(* Logix 5000 AddOnInstructionDefinition export Banner_IOL_Analog_Converter_Param_v4; software revision 33.00 *)

TYPE Banner_Analog_Converter_Port_Mirroringv4 :
STRUCT
   Mirroring_Output_Enable : SINT;   // 0 = Disabled, 1 = Enabled.
   Mirroring_Input_Port_Selection : SINT;   // 0 = Analog In 1, 1 = Analog In 2.
END_STRUCT
END_TYPE

TYPE Banner_Analog_Converter_RD_v4 :   // All of the read parameters for a S15C-I, S15C-U, R45-K-IQ, R45-K-UQ, R45C-KUU-UUQ, or R45C-KII-IIQ.
STRUCT
   Master_Cycle_Time : INT;
   Min_Cycle_Time : INT;
   M_Sequence_Capability : INT;
   IO_Link_Version_ID : INT;
   Process_Data_Input_Length : INT;
   Process_Data_Output_Length : INT;
   Combined_Vendor_ID : DINT;   // IO-Link Vendor ID
   Vendor_ID1 : INT;
   Vendor_ID2 : INT;
   Combined_Device_ID : DINT;   // IO-Link Device ID
   Device_ID1 : INT;
   Device_ID2 : INT;
   Device_ID3 : INT;
   Serial_Number : STRING;
   Product_Name : STRING;
   All_Time_Run_Time : DINT;   // Current All Time Run Timer.
   Model_Type : SINT;   // 0 = Voltage, 1 = Current
   MDC : Banner_MDC_Descriptor_v4[3];   // Array 0 not used. Array 1 is used for all models. Array 2 used for R45C Analog Double models.
END_STRUCT
END_TYPE

TYPE Banner_Analog_Converter_v4 :   // All of the parameters for a S15C-I, S15C-U, R45-K-IQ, R45-K-UQ, R45C-KUU-UUQ, or R45C-KII-IIQ.
STRUCT
   Initial_Global_Read : BOOL;   // Determines if all of the IO-Link data has been read into the PLC yet
   Command : INT;   // Value placed in here will activate a read or write to a specifc IO-Link Index
   Read : Banner_Analog_Converter_RD_v4;   // Read Only Data
   Write : Banner_Analog_Converter_WD_v4;   // Write Data
   Archive : Banner_Analog_Converter_WD_v4;   // Archive Data
   Reset : BOOL;   // Resets AOI. This will force a complete parameter read of the sensor.
END_STRUCT
END_TYPE

TYPE Banner_Analog_Converter_VSC_v4 :   // Vendor Specific Configuration data.
STRUCT
   PDI_Configuration : INT;   // 0 = Analog Value, 1 = Digital Measuring Sensor
   IOL_Filter_Time : DINT;   // Time to average IOL Process Data management between updates.
   PDO_Outside_Valid_Range : SINT;   // R45C-IU models only. 0 = Hold, 1 = Low, 2 = High.
   SSC1_PDO_Outside_Valid_Range : SINT;   // R45C Double Analog Models. 0 = Hold, 1 = Low, 2 = High.
   SSC2_PDO_Outside_Valid_Range : SINT;   // R45C Double Analog Models. 0 = Hold, 1 = Low, 2 = High.
   Secondary_Output_Function : SINT;   // R45C Double Analog Models. 0 = Disabled, 1 = Pulse Frequency Modulation.
   PFM_Input_Port : SINT;   // R45C Double Analog Models. 0 = Analog In1, 1 = Analog In 2.
END_STRUCT
END_TYPE

TYPE Banner_Analog_Converter_WD_v4 :   // UDT that stores the Write Data for a S15C-I, S15C-U, R45-K-IQ, R45-K-UQ, R45C-KUU-UUQ, or R45C-KII-IIQ.
STRUCT
   System_Command : INT;   // See IODD file for list of commands that can be activated via the System Command interface
   Parameter_Access_Lock : SINT;   // Write access to all parameters is prohibited while value is 1. Only this parameter can be adjusted when value is 1.
   Data_Storage_Lock : SINT;   // Automatic data storage is disabled when this value is equal to 1. Read access is not affected.
   Local_Parameterization_Lock : SINT;   // Parameterization via local control elements on device is disabled.
   Local_User_Interface_Lock : SINT;   // Operation of local user interface is disabled.
   BDC_Parameters : Banner_BDC_Parameters_v4[3];
   Port_Mirroring : Banner_Analog_Converter_Port_Mirroringv4[3];   // Only Double Analog Models.
   Resetable_Run_Time : DINT;   // Current Resetable Run Timer.
   VSC : Banner_Analog_Converter_VSC_v4;   // Vendor Specifc Configuration.
   All_Time_Run_Time_Event_Time : DINT;   // Time before an Event is generated. 0 = disable all-time event.
   Resetable_Run_Time_Event_Time : DINT;   // Time before an Event is generated. 0 = disable run time event.
   Pulse_Frequency : Banner_Pulse_Frequency_v4;
END_STRUCT
END_TYPE

TYPE Banner_BDC_Parameters_v4 :
STRUCT
   Setpoint_SP1 : DINT;
   Setpoint_SP2 : DINT;
   Switchpoint_Logic : SINT;   // 0 = Light Operate - Discrete Output is On while target detected.
   BDC_Mode : SINT;   // 2 = Window Mode. Defines how the binary switching information is created depending on Setpoint parameters and the current measurement value.
   Hysteresis : INT;   // Hysteresis value for the switchpoint.
END_STRUCT
END_TYPE

TYPE Banner_IOL_Port_v4 :   // UDT that has all of the data items necessary to communicate with a specific Port on a IO-Link Master
STRUCT
   Port_Controlled : INT;   // Each bit represents a port on an IO-Link Master. Set to 1 to tell AOI to control that port.
   Port_Activate : INT;   // Each bit represents a port on an IO-Link Master. When ON that port will process any commands in queue.
   Port_Read : INT;   // Each bit represents a port on an IO-Link Master. Used to determine when device AOI has requested a Read command.
   Port_Write : INT;   // Each bit represents a port on an IO-Link Master. Used to determine when device AOI has requested a Write command.
   Port_RW_Complete : INT;   // Each bit represents a port on an IO-Link Master. Tells device AOI that Read or Write request has been completed.
   Port_Device_Read : INT;
   Data_Transfer : SINT[190];   // Array to transfer data from IO-Master to device AOIs.
END_STRUCT
END_TYPE

TYPE Banner_MDC_Descriptor_v4 :
STRUCT
   Lower_Limit : DINT;
   Upper_Limit : DINT;
   Unit : DINT;   // 1209 = A, 1240 = V
   Scale : DINT;   // 260 = microAmps, 253 = microVolts
END_STRUCT
END_TYPE

TYPE Banner_Pulse_Frequency_v4 :   // Data items related to Pulse Frequency.
STRUCT
   Near_Frequency : DINT;   // 100 to 45000. Frequency corresponding to a target at the near limit of the sensing range.
   Far_Frequency : DINT;   // 100 to 45000. Frequency corresponding to a target at the far limit of the sensing range.
   Pulse_Frequenc_LOS : DINT;   // 50 to 45000. The frequency used to indicate loss of signal.
END_STRUCT
END_TYPE

ADD_ON_INSTRUCTION Banner_IOL_Analog_Converter_Param_v4   (* revision 4.0, vendor Banner Engineering *)
// AOI to read and write parameter data to an IO-Link S15C-I, S15C-U, R45-K-IQ, R45-K-UQ, R45C-KUU-UUQ, or R45C-KII-IIQ.
VAR_IN_OUT
   Converter : Banner_Analog_Converter_v4; {required}
   Port_Data : Banner_IOL_Port_v4; {required}
END_VAR
VAR_INPUT
   Port : DINT; {required}
   Type : DINT; {required}   // 0 for S15C U/I models. 1 for R45C U/I models. 2 for R45C UU/II double analog models.
END_VAR
VAR
   Local_Control : DINT; {access None}
   Global_Read_Command_Value : INT; {access None}
   Global_Write_Command_Value : INT; {access None}
   Error_Generated : BOOL; {access None}
   Command_Being_Processed : BOOL; {access None}
   Index_Write_Inprocess : INT; {access None}
   Index_Write_Control : INT; {access None}
   Update_Archive : BOOL; {access None}
   Inprocess_Index : DINT; {access None}
   Index : DINT; {access None}
   Index2 : DINT; {access None}
   Index3 : DINT; {access None}
END_VAR

ROUTINE Logic   (* ladder *)
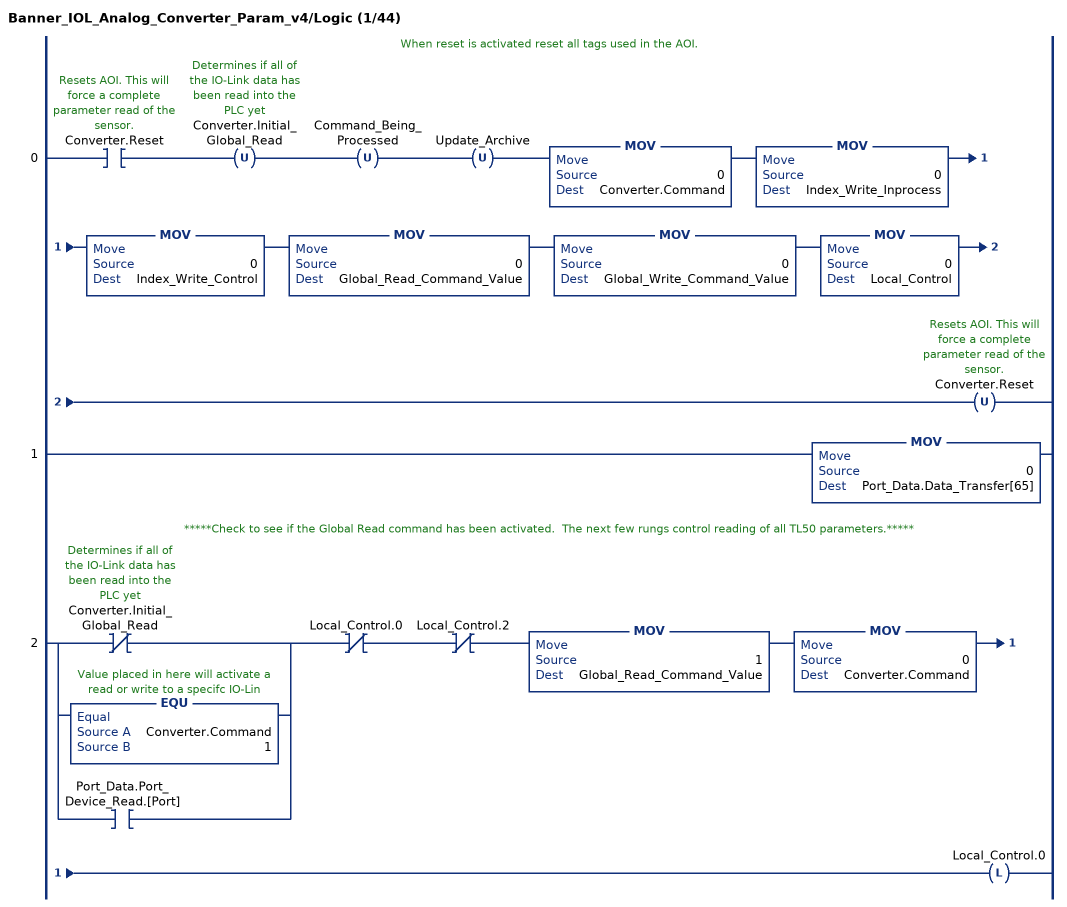
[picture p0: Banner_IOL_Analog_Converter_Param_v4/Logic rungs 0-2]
   // When reset is activated reset all tags used in the AOI.
   0: XIC(Converter.Reset)OTU(Converter.Initial_Global_Read)OTU(Command_Being_Processed)OTU(Update_Archive)MOV(0,Converter.Command)MOV(0,Index_Write_Inprocess)MOV(0,Index_Write_Control)MOV(0,Global_Read_Command_Value)MOV(0,Global_Write_Command_Value)MOV(0,Local_Control)OTU(Converter.Reset);
   1: MOV(0,Port_Data.Data_Transfer[65]);
   // *****Check to see if the Global Read command has been activated.  The next few rungs control reading of all TL50 parameters.*****
   2: [XIO(Converter.Initial_Global_Read) ,EQU(Converter.Command,1) ,XIC(Port_Data.Port_Device_Read.[Port]) ]XIO(Local_Control.0)XIO(Local_Control.2)MOV(1,Global_Read_Command_Value)MOV(0,Converter.Command)OTL(Local_Control.0);
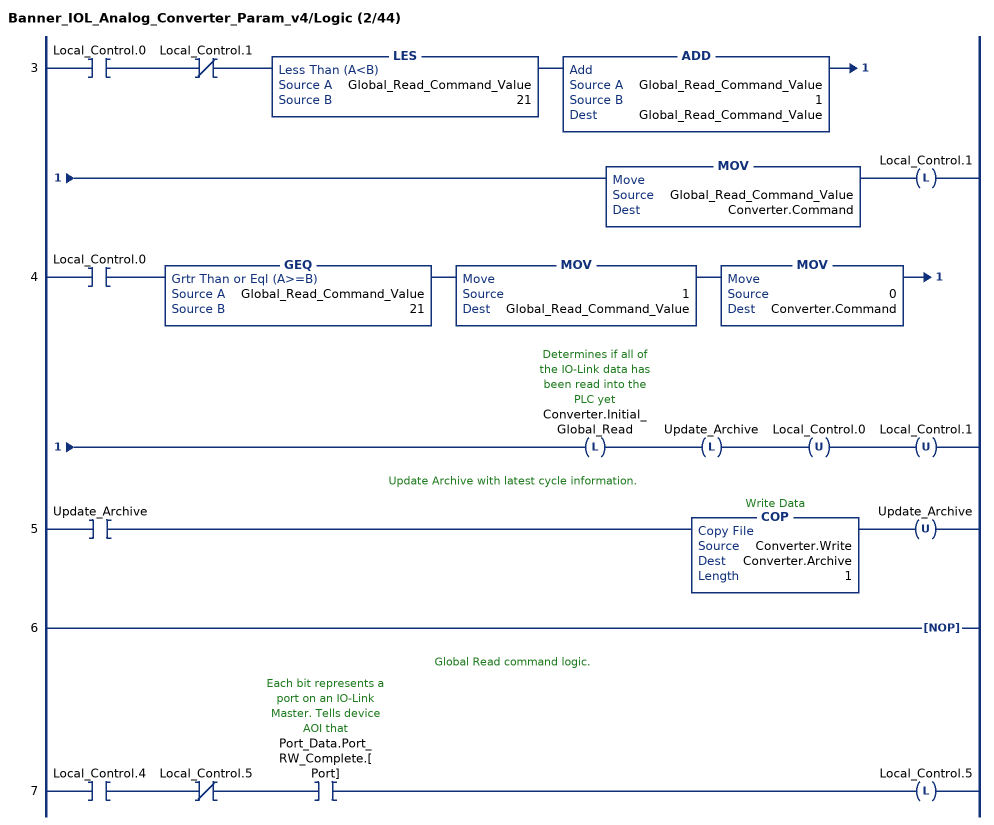
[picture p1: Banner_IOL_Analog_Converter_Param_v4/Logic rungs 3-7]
   3: XIC(Local_Control.0)XIO(Local_Control.1)LES(Global_Read_Command_Value,21)ADD(Global_Read_Command_Value,1,Global_Read_Command_Value)MOV(Global_Read_Command_Value,Converter.Command)OTL(Local_Control.1);
   4: XIC(Local_Control.0)GEQ(Global_Read_Command_Value,21)MOV(1,Global_Read_Command_Value)MOV(0,Converter.Command)OTL(Converter.Initial_Global_Read)OTL(Update_Archive)OTU(Local_Control.0)OTU(Local_Control.1);
   // Update Archive with latest cycle information.
   5: XIC(Update_Archive)COP(Converter.Write,Converter.Archive,1)OTU(Update_Archive);
   6: NOP();
   // Global Read command logic.
   7: XIC(Local_Control.4)XIO(Local_Control.5)XIC(Port_Data.Port_RW_Complete.[Port])OTL(Local_Control.5);
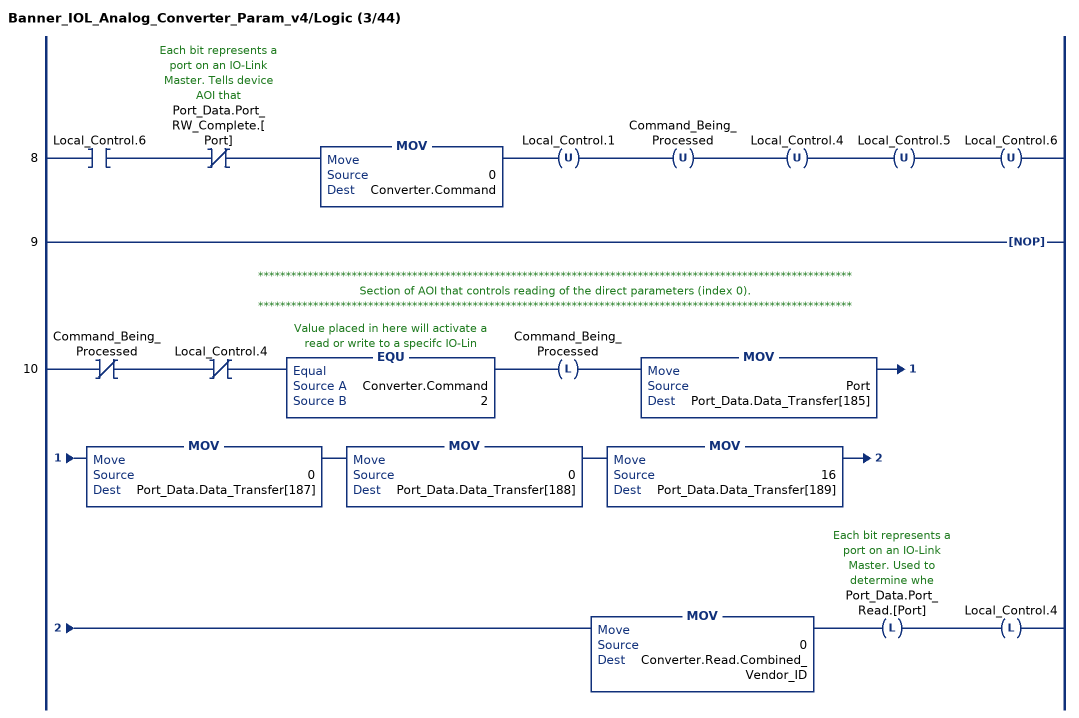
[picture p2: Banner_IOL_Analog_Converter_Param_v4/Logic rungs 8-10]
   8: XIC(Local_Control.6)XIO(Port_Data.Port_RW_Complete.[Port])MOV(0,Converter.Command)OTU(Local_Control.1)OTU(Command_Being_Processed)OTU(Local_Control.4)OTU(Local_Control.5)OTU(Local_Control.6);
   9: NOP();
   // ************************************************************************************************************
   // Section of AOI that controls reading of the direct parameters (index 0).
   // ************************************************************************************************************
   10: XIO(Command_Being_Processed)XIO(Local_Control.4)EQU(Converter.Command,2)OTL(Command_Being_Processed)MOV(Port,Port_Data.Data_Transfer[185])MOV(0,Port_Data.Data_Transfer[187])MOV(0,Port_Data.Data_Transfer[188])MOV(16,Port_Data.Data_Transfer[189])MOV(0,Converter.Read.Combined_Vendor_ID)OTL(Port_Data.Port_Read.[Port])OTL(Local_Control.4);
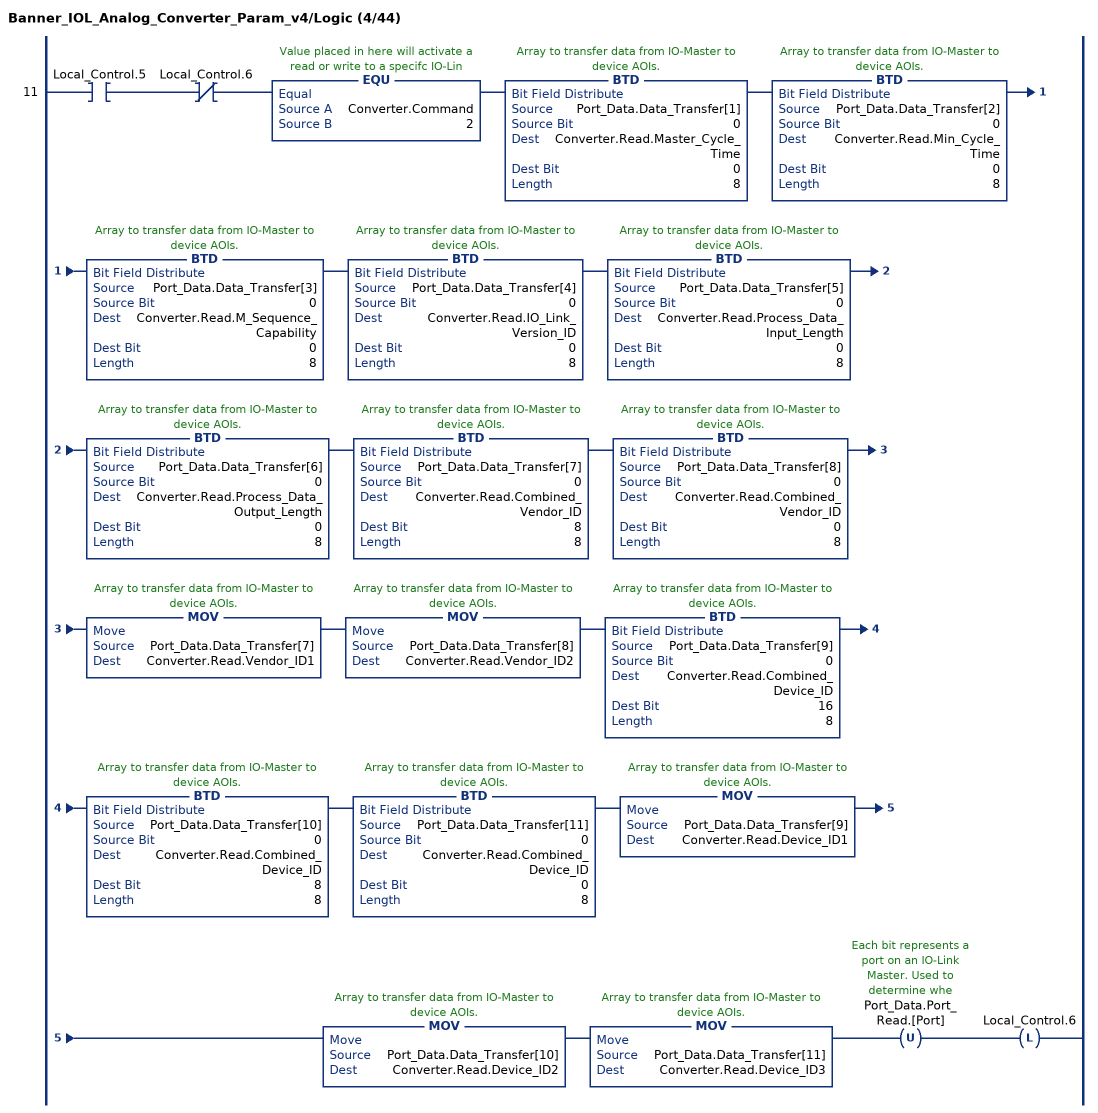
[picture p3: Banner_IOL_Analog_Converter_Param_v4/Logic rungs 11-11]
   11: XIC(Local_Control.5)XIO(Local_Control.6)EQU(Converter.Command,2)BTD(Port_Data.Data_Transfer[1],0,Converter.Read.Master_Cycle_Time,0,8)BTD(Port_Data.Data_Transfer[2],0,Converter.Read.Min_Cycle_Time,0,8)BTD(Port_Data.Data_Transfer[3],0,Converter.Read.M_Sequence_Capability,0,8)BTD(Port_Data.Data_Transfer[4],0,Converter.Read.IO_Link_Version_ID,0,8)BTD(Port_Data.Data_Transfer[5],0,Converter.Read.Process_Data_Input_Length,0,8)BTD(Port_Data.Data_Transfer[6],0,Converter.Read.Process_Data_Output_Length,0,8)BTD(Port_Data.Data_Transfer[7],0,Converter.Read.Combined_Vendor_ID,8,8)BTD(Port_Data.Data_Transfer[8],0,Converter.Read.Combined_Vendor_ID,0,8)MOV(Port_Data.Data_Transfer[7],Converter.Read.Vendor_ID1)MOV(Port_Data.Data_Transfer[8],Converter.Read.Vendor_ID2)BTD(Port_Data.Data_Transfer[9],0,Converter.Read.Combined_Device_ID,16,8)BTD(Port_Data.Data_Transfer[10],0,Converter.Read.Combined_Device_ID,8,8)BTD(Port_Data.Data_Transfer[11],0,Converter.Read.Combined_Device_ID,0,8)MOV(Port_Data.Data_Transfer[9],Converter.Read.Device_ID1)MOV(Port_Data.Data_Transfer[10],Converter.Read.Device_ID2)MOV(Port_Data.Data_Transfer[11],Converter.Read.Device_ID3)OTU(Port_Data.Port_Read.[Port])OTL(Local_Control.6);
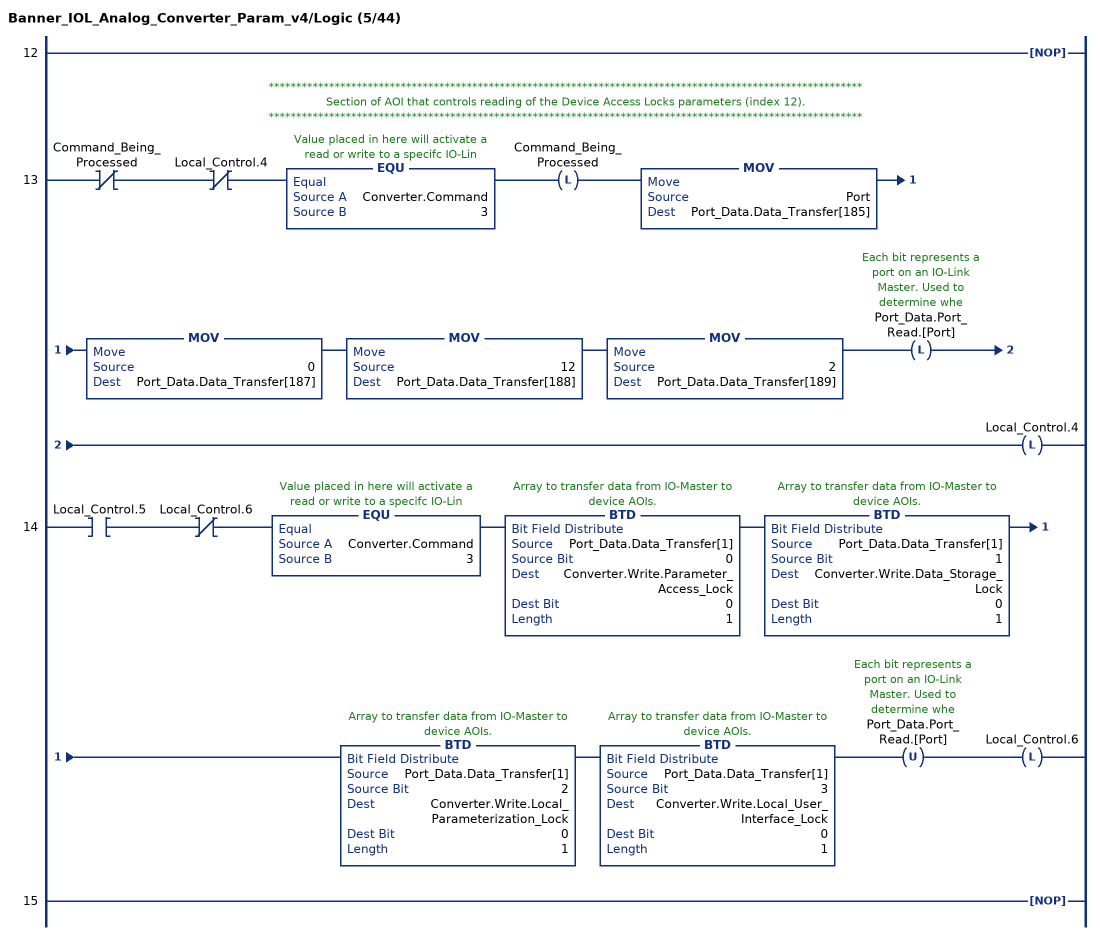
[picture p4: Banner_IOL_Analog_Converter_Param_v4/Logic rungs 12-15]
   12: NOP();
   // ************************************************************************************************************
   // Section of AOI that controls reading of the Device Access Locks parameters (index 12).
   // ************************************************************************************************************
   13: XIO(Command_Being_Processed)XIO(Local_Control.4)EQU(Converter.Command,3)OTL(Command_Being_Processed)MOV(Port,Port_Data.Data_Transfer[185])MOV(0,Port_Data.Data_Transfer[187])MOV(12,Port_Data.Data_Transfer[188])MOV(2,Port_Data.Data_Transfer[189])OTL(Port_Data.Port_Read.[Port])OTL(Local_Control.4);
   14: XIC(Local_Control.5)XIO(Local_Control.6)EQU(Converter.Command,3)BTD(Port_Data.Data_Transfer[1],0,Converter.Write.Parameter_Access_Lock,0,1)BTD(Port_Data.Data_Transfer[1],1,Converter.Write.Data_Storage_Lock,0,1)BTD(Port_Data.Data_Transfer[1],2,Converter.Write.Local_Parameterization_Lock,0,1)BTD(Port_Data.Data_Transfer[1],3,Converter.Write.Local_User_Interface_Lock,0,1)OTU(Port_Data.Port_Read.[Port])OTL(Local_Control.6);
   15: NOP();
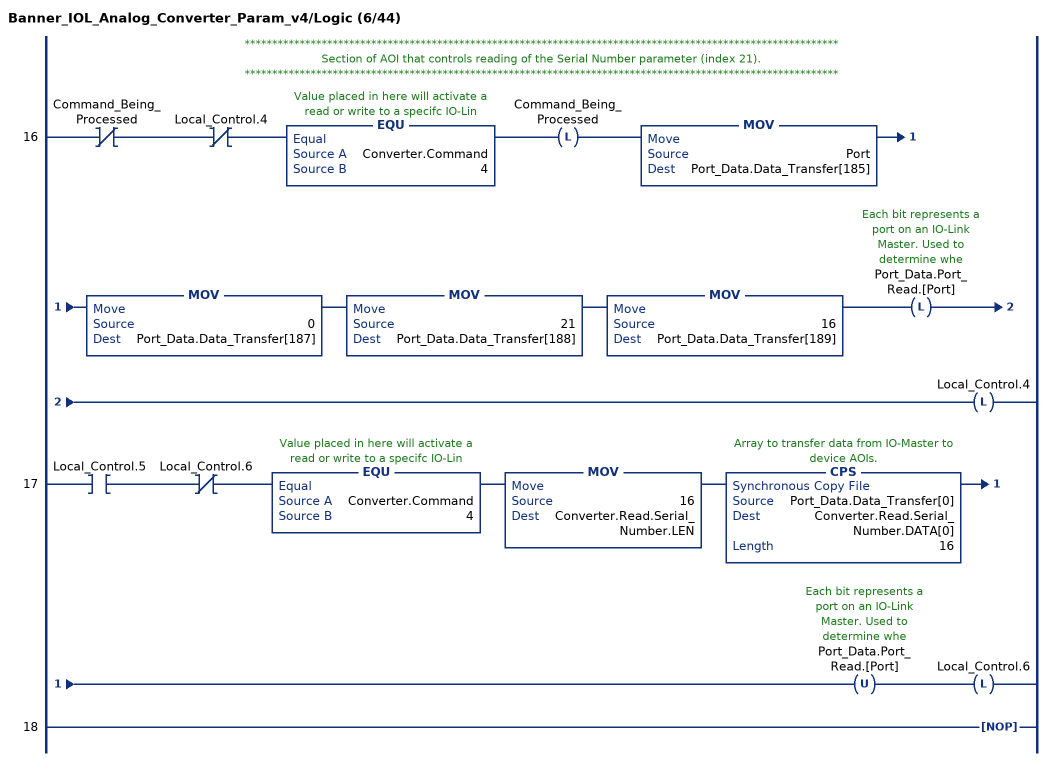
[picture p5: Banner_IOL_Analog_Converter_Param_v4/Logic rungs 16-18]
   // ************************************************************************************************************
   // Section of AOI that controls reading of the Serial Number parameter (index 21).
   // ************************************************************************************************************
   16: XIO(Command_Being_Processed)XIO(Local_Control.4)EQU(Converter.Command,4)OTL(Command_Being_Processed)MOV(Port,Port_Data.Data_Transfer[185])MOV(0,Port_Data.Data_Transfer[187])MOV(21,Port_Data.Data_Transfer[188])MOV(16,Port_Data.Data_Transfer[189])OTL(Port_Data.Port_Read.[Port])OTL(Local_Control.4);
   17: XIC(Local_Control.5)XIO(Local_Control.6)EQU(Converter.Command,4)MOV(16,Converter.Read.Serial_Number.LEN)CPS(Port_Data.Data_Transfer[0],Converter.Read.Serial_Number.DATA[0],16)OTU(Port_Data.Port_Read.[Port])OTL(Local_Control.6);
   18: NOP();
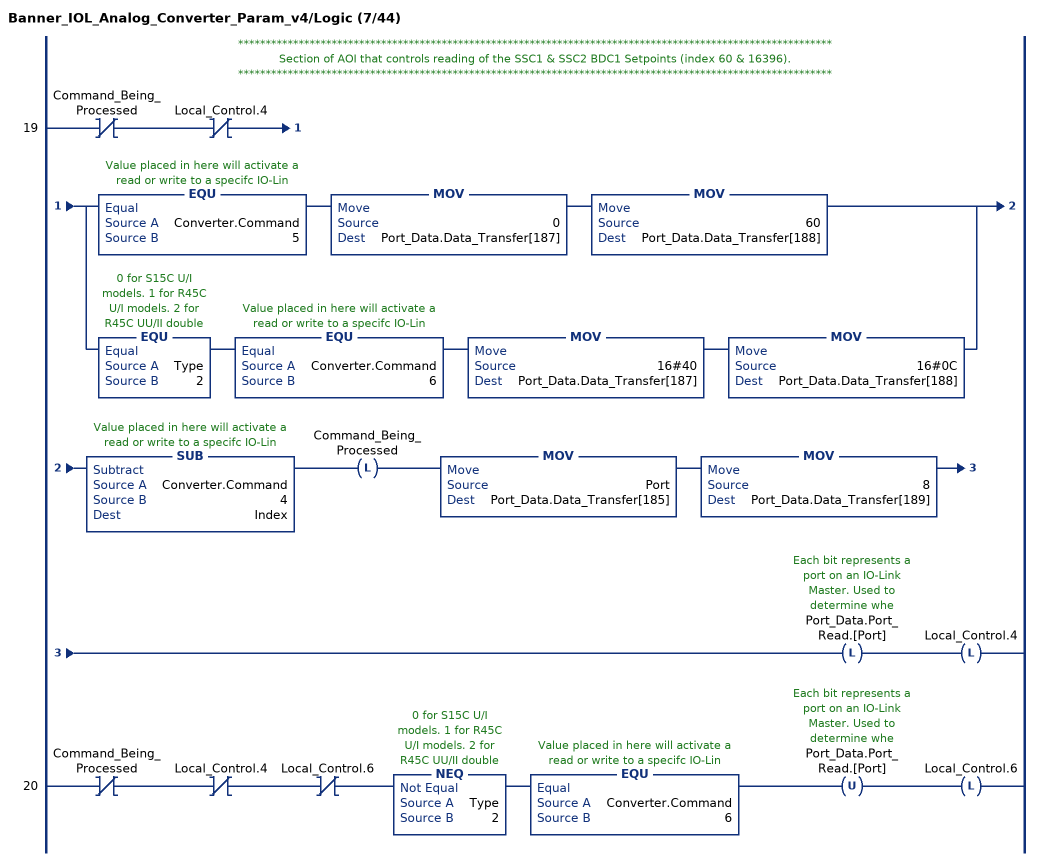
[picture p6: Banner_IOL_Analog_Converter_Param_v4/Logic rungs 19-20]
   // ************************************************************************************************************
   // Section of AOI that controls reading of the SSC1 & SSC2 BDC1 Setpoints (index 60 & 16396).
   // ************************************************************************************************************
   19: XIO(Command_Being_Processed)XIO(Local_Control.4)[EQU(Converter.Command,5) MOV(0,Port_Data.Data_Transfer[187]) MOV(60,Port_Data.Data_Transfer[188]) ,EQU(Type,2) EQU(Converter.Command,6) MOV(16#40,Port_Data.Data_Transfer[187]) MOV(16#0C,Port_Data.Data_Transfer[188]) ]SUB(Converter.Command,4,Index)OTL(Command_Being_Processed)MOV(Port,Port_Data.Data_Transfer[185])MOV(8,Port_Data.Data_Transfer[189])OTL(Port_Data.Port_Read.[Port])OTL(Local_Control.4);
   20: XIO(Command_Being_Processed)XIO(Local_Control.4)XIO(Local_Control.6)NEQ(Type,2)EQU(Converter.Command,6)OTU(Port_Data.Port_Read.[Port])OTL(Local_Control.6);
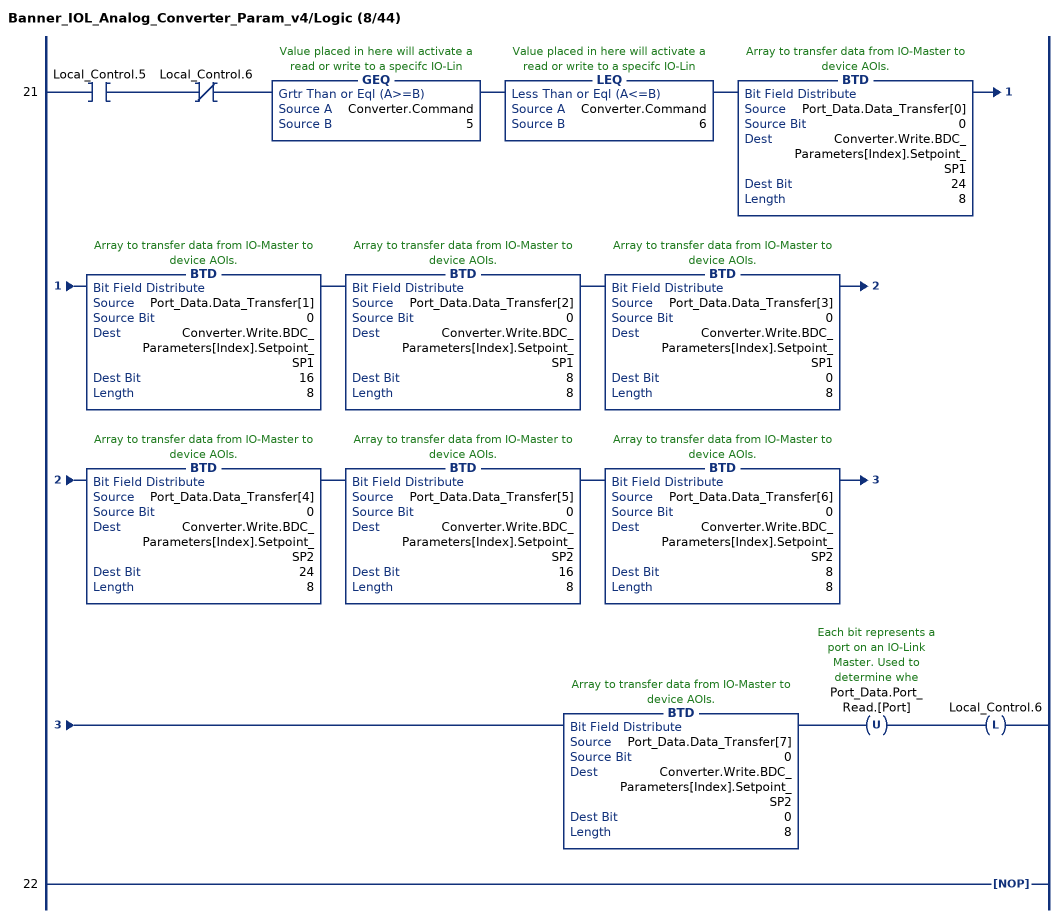
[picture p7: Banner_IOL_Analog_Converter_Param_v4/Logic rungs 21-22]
   21: XIC(Local_Control.5)XIO(Local_Control.6)GEQ(Converter.Command,5)LEQ(Converter.Command,6)BTD(Port_Data.Data_Transfer[0],0,Converter.Write.BDC_Parameters[Index].Setpoint_SP1,24,8)BTD(Port_Data.Data_Transfer[1],0,Converter.Write.BDC_Parameters[Index].Setpoint_SP1,16,8)BTD(Port_Data.Data_Transfer[2],0,Converter.Write.BDC_Parameters[Index].Setpoint_SP1,8,8)BTD(Port_Data.Data_Transfer[3],0,Converter.Write.BDC_Parameters[Index].Setpoint_SP1,0,8)BTD(Port_Data.Data_Transfer[4],0,Converter.Write.BDC_Parameters[Index].Setpoint_SP2,24,8)BTD(Port_Data.Data_Transfer[5],0,Converter.Write.BDC_Parameters[Index].Setpoint_SP2,16,8)BTD(Port_Data.Data_Transfer[6],0,Converter.Write.BDC_Parameters[Index].Setpoint_SP2,8,8)BTD(Port_Data.Data_Transfer[7],0,Converter.Write.BDC_Parameters[Index].Setpoint_SP2,0,8)OTU(Port_Data.Port_Read.[Port])OTL(Local_Control.6);
   22: NOP();
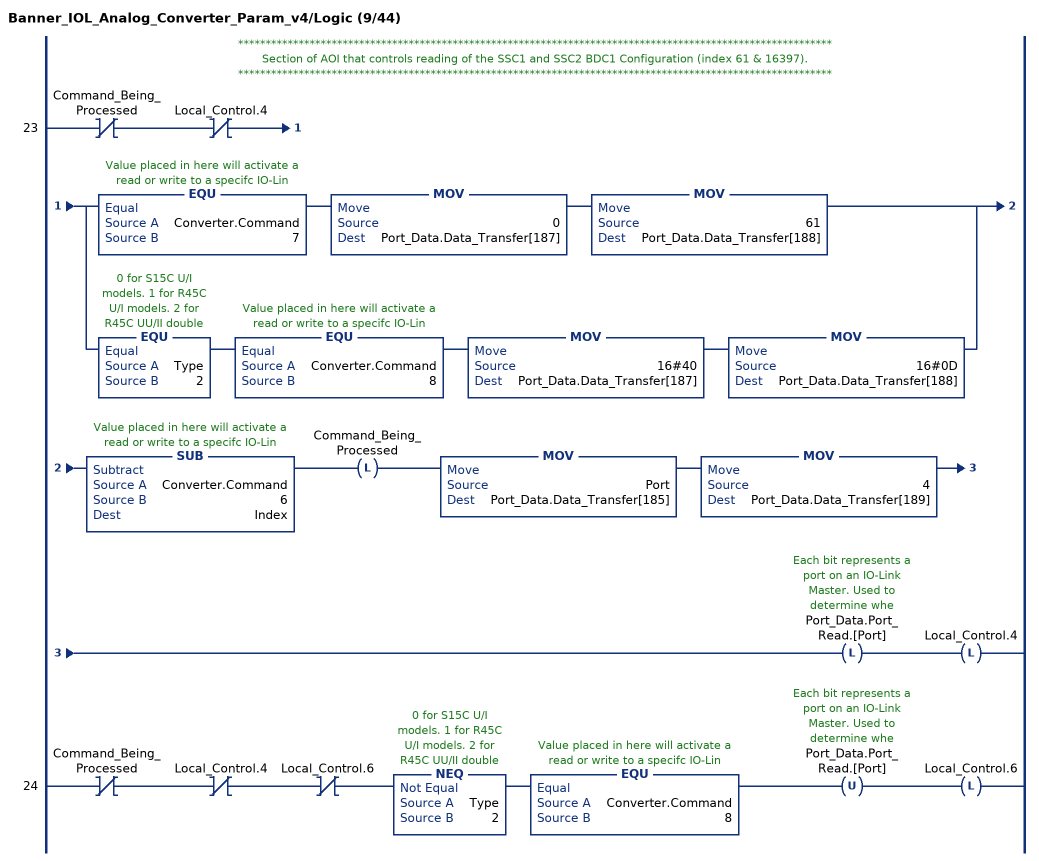
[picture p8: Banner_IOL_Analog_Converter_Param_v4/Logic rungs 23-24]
   // ************************************************************************************************************
   // Section of AOI that controls reading of the SSC1 and SSC2 BDC1 Configuration (index 61 & 16397).
   // ************************************************************************************************************
   23: XIO(Command_Being_Processed)XIO(Local_Control.4)[EQU(Converter.Command,7) MOV(0,Port_Data.Data_Transfer[187]) MOV(61,Port_Data.Data_Transfer[188]) ,EQU(Type,2) EQU(Converter.Command,8) MOV(16#40,Port_Data.Data_Transfer[187]) MOV(16#0D,Port_Data.Data_Transfer[188]) ]SUB(Converter.Command,6,Index)OTL(Command_Being_Processed)MOV(Port,Port_Data.Data_Transfer[185])MOV(4,Port_Data.Data_Transfer[189])OTL(Port_Data.Port_Read.[Port])OTL(Local_Control.4);
   24: XIO(Command_Being_Processed)XIO(Local_Control.4)XIO(Local_Control.6)NEQ(Type,2)EQU(Converter.Command,8)OTU(Port_Data.Port_Read.[Port])OTL(Local_Control.6);
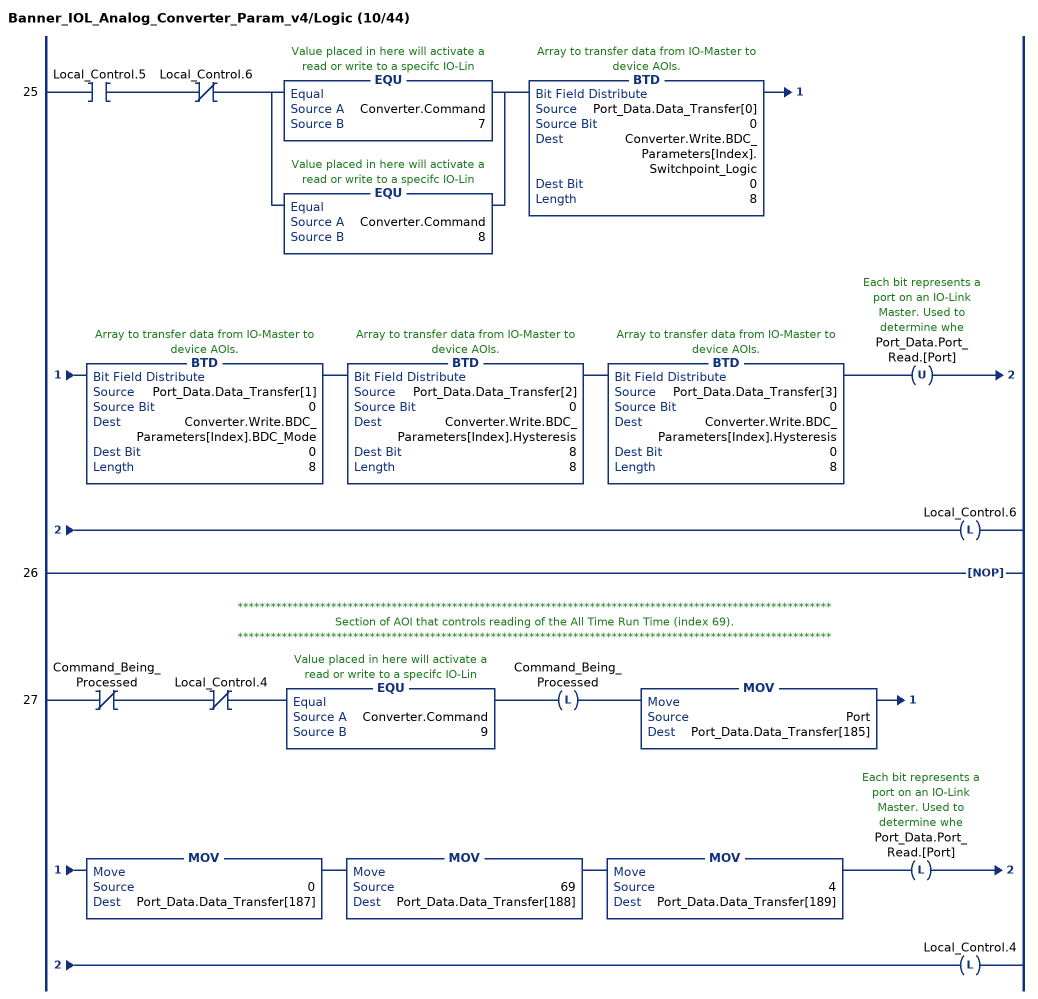
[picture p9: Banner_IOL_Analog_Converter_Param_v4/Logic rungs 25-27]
   25: XIC(Local_Control.5)XIO(Local_Control.6)[EQU(Converter.Command,7) ,EQU(Converter.Command,8) ]BTD(Port_Data.Data_Transfer[0],0,Converter.Write.BDC_Parameters[Index].Switchpoint_Logic,0,8)BTD(Port_Data.Data_Transfer[1],0,Converter.Write.BDC_Parameters[Index].BDC_Mode,0,8)BTD(Port_Data.Data_Transfer[2],0,Converter.Write.BDC_Parameters[Index].Hysteresis,8,8)BTD(Port_Data.Data_Transfer[3],0,Converter.Write.BDC_Parameters[Index].Hysteresis,0,8)OTU(Port_Data.Port_Read.[Port])OTL(Local_Control.6);
   26: NOP();
   // ************************************************************************************************************
   // Section of AOI that controls reading of the All Time Run Time (index 69).
   // ************************************************************************************************************
   27: XIO(Command_Being_Processed)XIO(Local_Control.4)EQU(Converter.Command,9)OTL(Command_Being_Processed)MOV(Port,Port_Data.Data_Transfer[185])MOV(0,Port_Data.Data_Transfer[187])MOV(69,Port_Data.Data_Transfer[188])MOV(4,Port_Data.Data_Transfer[189])OTL(Port_Data.Port_Read.[Port])OTL(Local_Control.4);
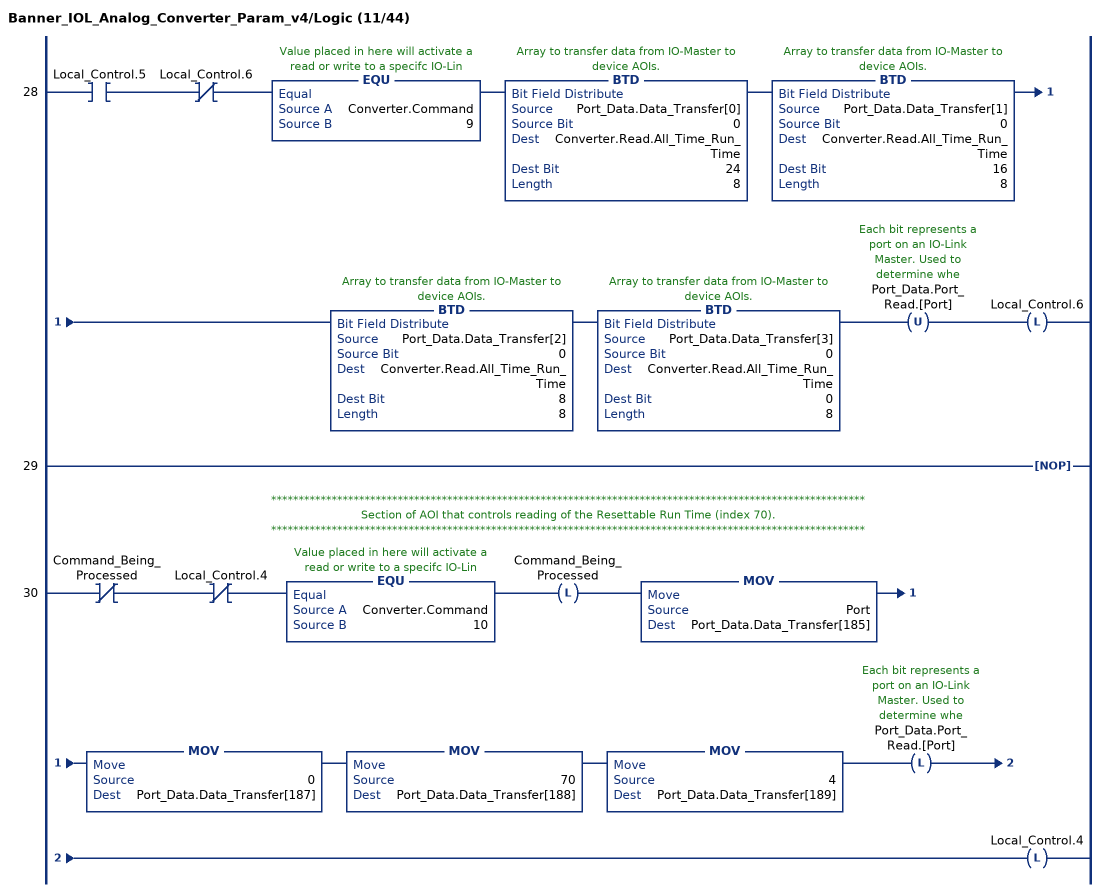
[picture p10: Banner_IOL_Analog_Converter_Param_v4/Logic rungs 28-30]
   28: XIC(Local_Control.5)XIO(Local_Control.6)EQU(Converter.Command,9)BTD(Port_Data.Data_Transfer[0],0,Converter.Read.All_Time_Run_Time,24,8)BTD(Port_Data.Data_Transfer[1],0,Converter.Read.All_Time_Run_Time,16,8)BTD(Port_Data.Data_Transfer[2],0,Converter.Read.All_Time_Run_Time,8,8)BTD(Port_Data.Data_Transfer[3],0,Converter.Read.All_Time_Run_Time,0,8)OTU(Port_Data.Port_Read.[Port])OTL(Local_Control.6);
   29: NOP();
   // ************************************************************************************************************
   // Section of AOI that controls reading of the Resettable Run Time (index 70).
   // ************************************************************************************************************
   30: XIO(Command_Being_Processed)XIO(Local_Control.4)EQU(Converter.Command,10)OTL(Command_Being_Processed)MOV(Port,Port_Data.Data_Transfer[185])MOV(0,Port_Data.Data_Transfer[187])MOV(70,Port_Data.Data_Transfer[188])MOV(4,Port_Data.Data_Transfer[189])OTL(Port_Data.Port_Read.[Port])OTL(Local_Control.4);
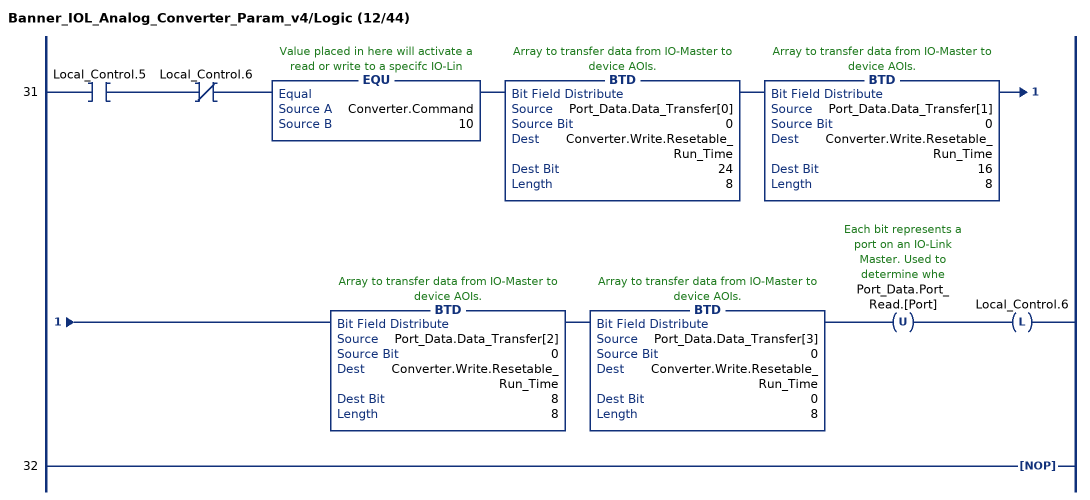
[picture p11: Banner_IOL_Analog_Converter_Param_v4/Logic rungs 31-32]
   31: XIC(Local_Control.5)XIO(Local_Control.6)EQU(Converter.Command,10)BTD(Port_Data.Data_Transfer[0],0,Converter.Write.Resetable_Run_Time,24,8)BTD(Port_Data.Data_Transfer[1],0,Converter.Write.Resetable_Run_Time,16,8)BTD(Port_Data.Data_Transfer[2],0,Converter.Write.Resetable_Run_Time,8,8)BTD(Port_Data.Data_Transfer[3],0,Converter.Write.Resetable_Run_Time,0,8)OTU(Port_Data.Port_Read.[Port])OTL(Local_Control.6);
   32: NOP();
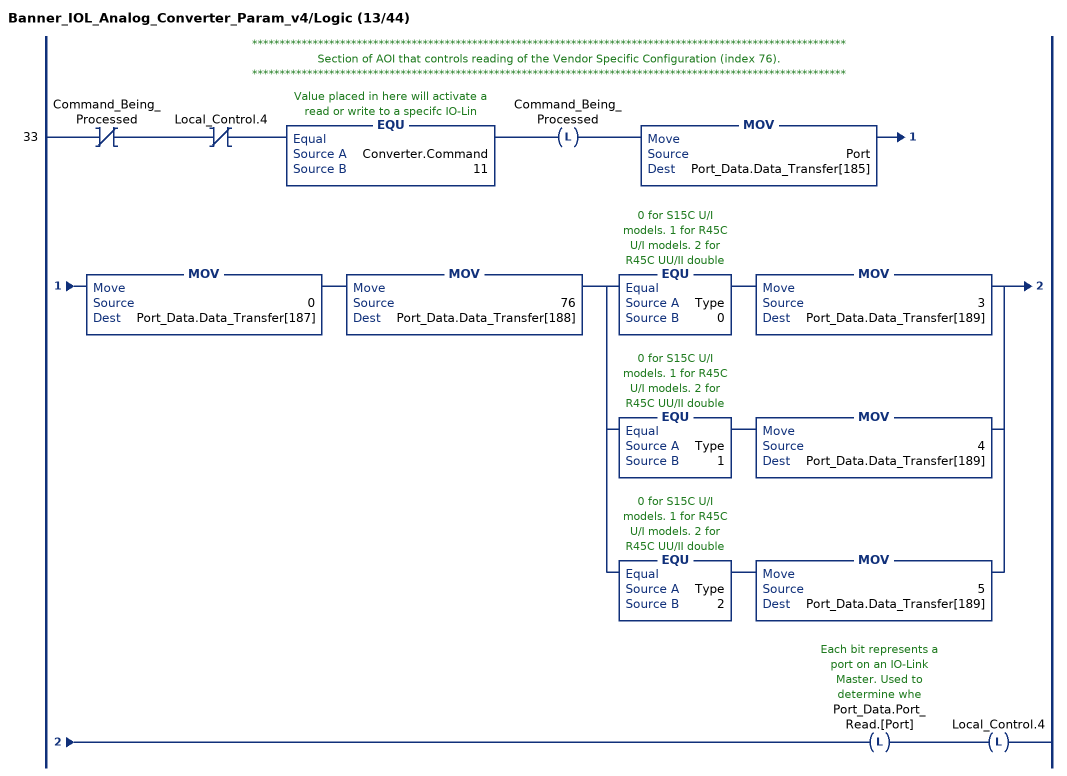
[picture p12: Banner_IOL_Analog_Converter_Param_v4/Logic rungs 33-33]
   // ************************************************************************************************************
   // Section of AOI that controls reading of the Vendor Specific Configuration (index 76).
   // ************************************************************************************************************
   33: XIO(Command_Being_Processed)XIO(Local_Control.4)EQU(Converter.Command,11)OTL(Command_Being_Processed)MOV(Port,Port_Data.Data_Transfer[185])MOV(0,Port_Data.Data_Transfer[187])MOV(76,Port_Data.Data_Transfer[188])[EQU(Type,0) MOV(3,Port_Data.Data_Transfer[189]) ,EQU(Type,1) MOV(4,Port_Data.Data_Transfer[189]) ,EQU(Type,2) MOV(5,Port_Data.Data_Transfer[189]) ]OTL(Port_Data.Port_Read.[Port])OTL(Local_Control.4);
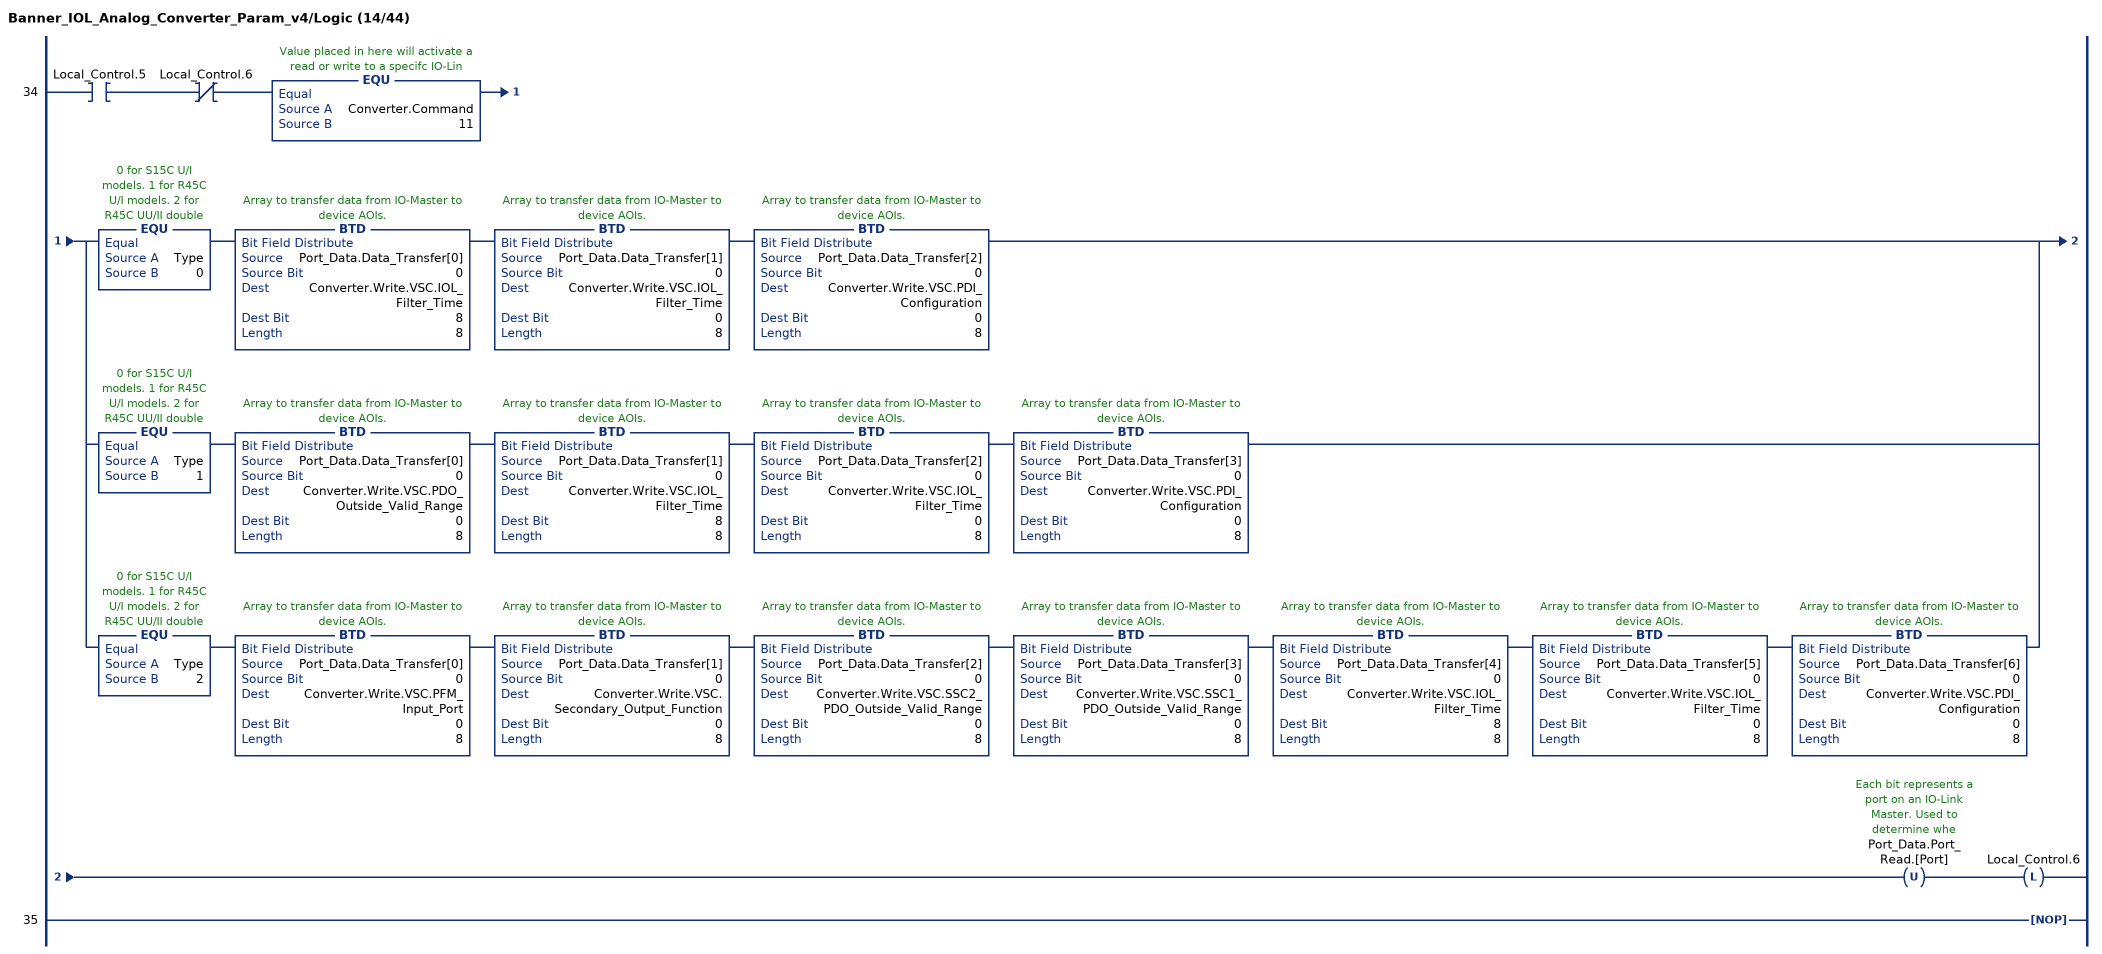
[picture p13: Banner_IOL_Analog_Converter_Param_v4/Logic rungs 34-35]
   34: XIC(Local_Control.5)XIO(Local_Control.6)EQU(Converter.Command,11)[EQU(Type,0) BTD(Port_Data.Data_Transfer[0],0,Converter.Write.VSC.IOL_Filter_Time,8,8) BTD(Port_Data.Data_Transfer[1],0,Converter.Write.VSC.IOL_Filter_Time,0,8) BTD(Port_Data.Data_Transfer[2],0,Converter.Write.VSC.PDI_Configuration,0,8) ,EQU(Type,1) BTD(Port_Data.Data_Transfer[0],0,Converter.Write.VSC.PDO_Outside_Valid_Range,0,8) BTD(Port_Data.Data_Transfer[1],0,Converter.Write.VSC.IOL_Filter_Time,8,8) BTD(Port_Data.Data_Transfer[2],0,Converter.Write.VSC.IOL_Filter_Time,0,8) BTD(Port_Data.Data_Transfer[3],0,Converter.Write.VSC.PDI_Configuration,0,8) ,EQU(Type,2) BTD(Port_Data.Data_Transfer[0],0,Converter.Write.VSC.PFM_Input_Port,0,8) BTD(Port_Data.Data_Transfer[1],0,Converter.Write.VSC.Secondary_Output_Function,0,8) BTD(Port_Data.Data_Transfer[2],0,Converter.Write.VSC.SSC2_PDO_Outside_Valid_Range,0,8) BTD(Port_Data.Data_Transfer[3],0,Converter.Write.VSC.SSC1_PDO_Outside_Valid_Range,0,8) BTD(Port_Data.Data_Transfer[4],0,Converter.Write.VSC.IOL_Filter_Time,8,8) BTD(Port_Data.Data_Transfer[5],0,Converter.Write.VSC.IOL_Filter_Time,0,8) BTD(Port_Data.Data_Transfer[6],0,Converter.Write.VSC.PDI_Configuration,0,8) ]OTU(Port_Data.Port_Read.[Port])OTL(Local_Control.6);
   35: NOP();
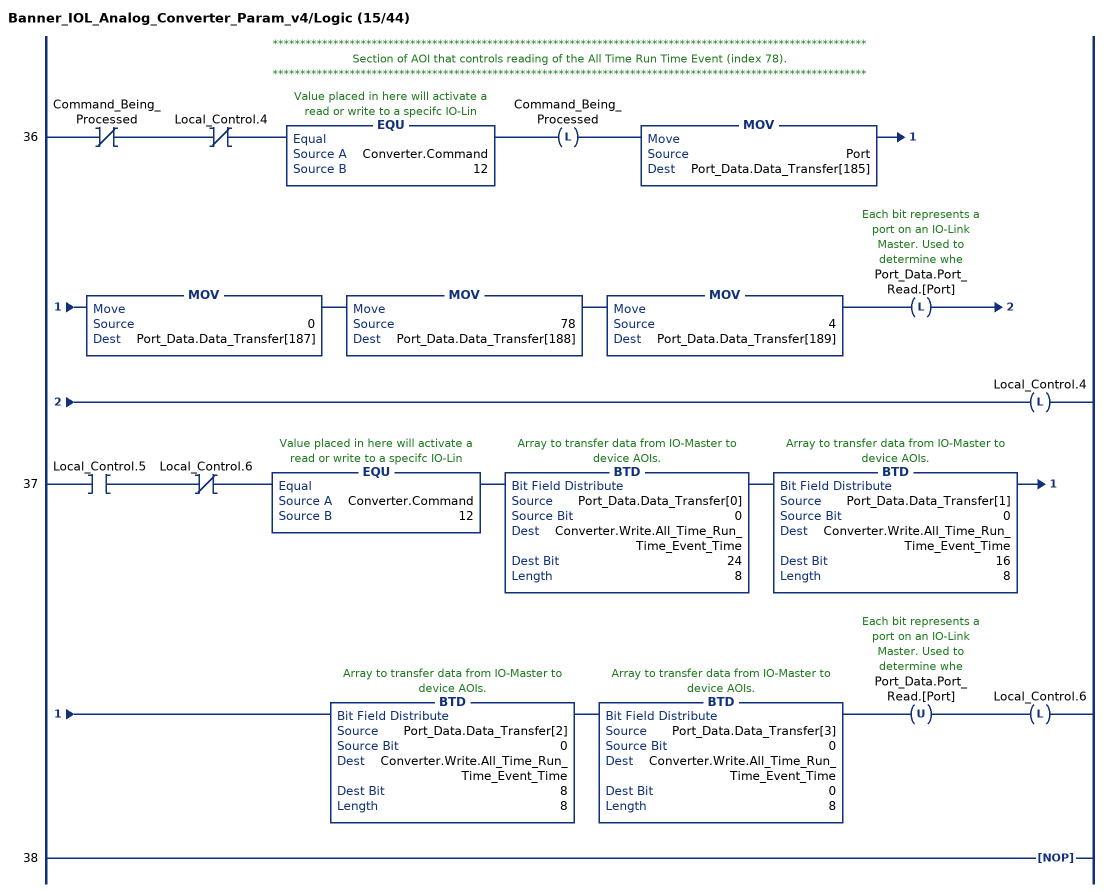
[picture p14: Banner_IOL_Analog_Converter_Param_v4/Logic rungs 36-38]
   // ************************************************************************************************************
   // Section of AOI that controls reading of the All Time Run Time Event (index 78).
   // ************************************************************************************************************
   36: XIO(Command_Being_Processed)XIO(Local_Control.4)EQU(Converter.Command,12)OTL(Command_Being_Processed)MOV(Port,Port_Data.Data_Transfer[185])MOV(0,Port_Data.Data_Transfer[187])MOV(78,Port_Data.Data_Transfer[188])MOV(4,Port_Data.Data_Transfer[189])OTL(Port_Data.Port_Read.[Port])OTL(Local_Control.4);
   37: XIC(Local_Control.5)XIO(Local_Control.6)EQU(Converter.Command,12)BTD(Port_Data.Data_Transfer[0],0,Converter.Write.All_Time_Run_Time_Event_Time,24,8)BTD(Port_Data.Data_Transfer[1],0,Converter.Write.All_Time_Run_Time_Event_Time,16,8)BTD(Port_Data.Data_Transfer[2],0,Converter.Write.All_Time_Run_Time_Event_Time,8,8)BTD(Port_Data.Data_Transfer[3],0,Converter.Write.All_Time_Run_Time_Event_Time,0,8)OTU(Port_Data.Port_Read.[Port])OTL(Local_Control.6);
   38: NOP();
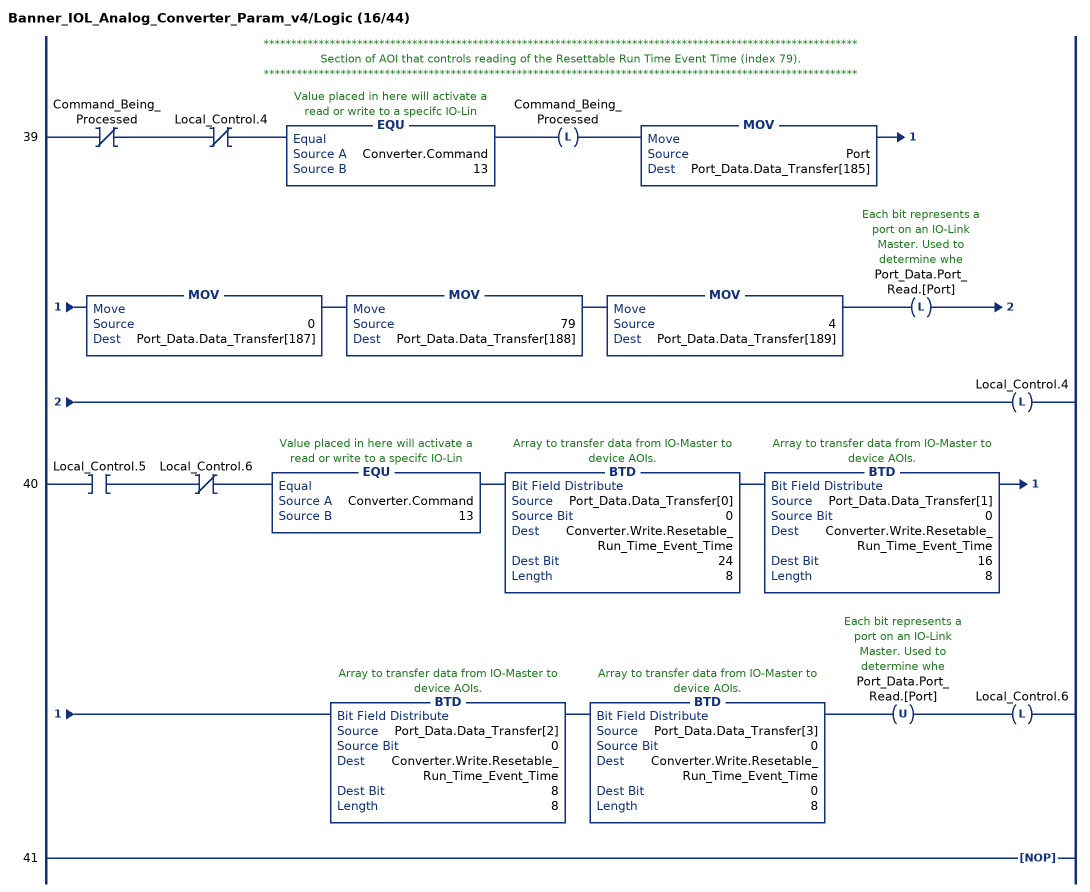
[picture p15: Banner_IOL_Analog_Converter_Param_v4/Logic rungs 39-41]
   // ************************************************************************************************************
   // Section of AOI that controls reading of the Resettable Run Time Event Time (index 79).
   // ************************************************************************************************************
   39: XIO(Command_Being_Processed)XIO(Local_Control.4)EQU(Converter.Command,13)OTL(Command_Being_Processed)MOV(Port,Port_Data.Data_Transfer[185])MOV(0,Port_Data.Data_Transfer[187])MOV(79,Port_Data.Data_Transfer[188])MOV(4,Port_Data.Data_Transfer[189])OTL(Port_Data.Port_Read.[Port])OTL(Local_Control.4);
   40: XIC(Local_Control.5)XIO(Local_Control.6)EQU(Converter.Command,13)BTD(Port_Data.Data_Transfer[0],0,Converter.Write.Resetable_Run_Time_Event_Time,24,8)BTD(Port_Data.Data_Transfer[1],0,Converter.Write.Resetable_Run_Time_Event_Time,16,8)BTD(Port_Data.Data_Transfer[2],0,Converter.Write.Resetable_Run_Time_Event_Time,8,8)BTD(Port_Data.Data_Transfer[3],0,Converter.Write.Resetable_Run_Time_Event_Time,0,8)OTU(Port_Data.Port_Read.[Port])OTL(Local_Control.6);
   41: NOP();
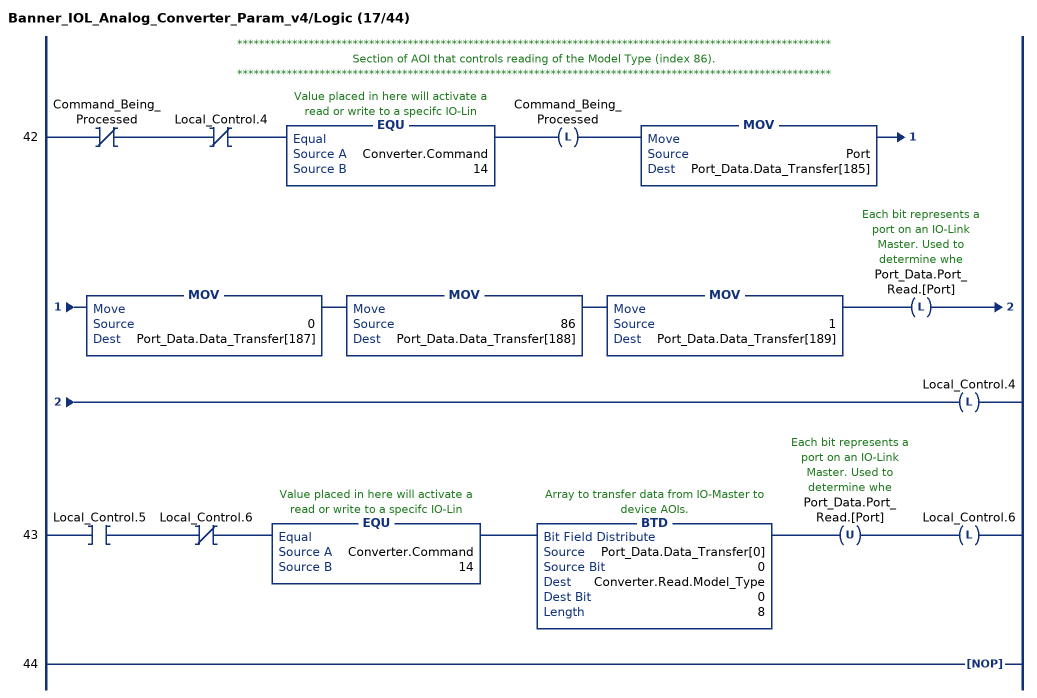
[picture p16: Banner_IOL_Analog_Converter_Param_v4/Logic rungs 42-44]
   // ************************************************************************************************************
   // Section of AOI that controls reading of the Model Type (index 86).
   // ************************************************************************************************************
   42: XIO(Command_Being_Processed)XIO(Local_Control.4)EQU(Converter.Command,14)OTL(Command_Being_Processed)MOV(Port,Port_Data.Data_Transfer[185])MOV(0,Port_Data.Data_Transfer[187])MOV(86,Port_Data.Data_Transfer[188])MOV(1,Port_Data.Data_Transfer[189])OTL(Port_Data.Port_Read.[Port])OTL(Local_Control.4);
   43: XIC(Local_Control.5)XIO(Local_Control.6)EQU(Converter.Command,14)BTD(Port_Data.Data_Transfer[0],0,Converter.Read.Model_Type,0,8)OTU(Port_Data.Port_Read.[Port])OTL(Local_Control.6);
   44: NOP();
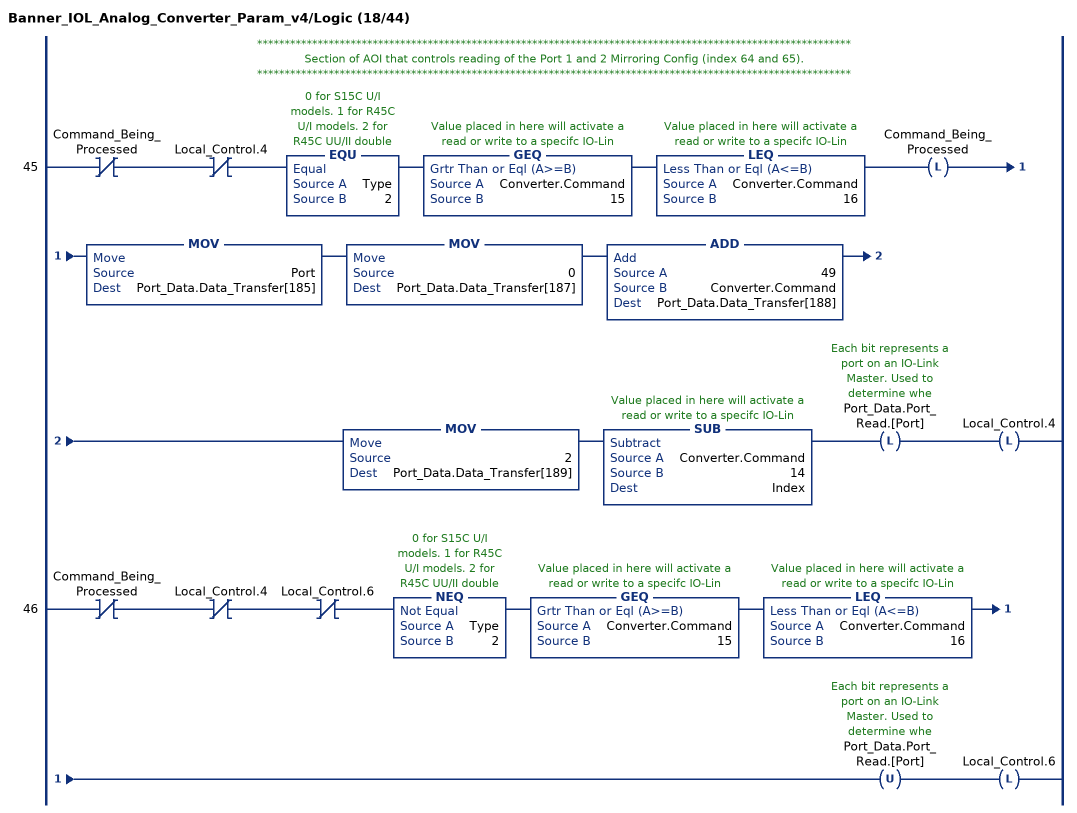
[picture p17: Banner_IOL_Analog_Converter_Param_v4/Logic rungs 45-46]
   // ************************************************************************************************************
   // Section of AOI that controls reading of the Port 1 and 2 Mirroring Config (index 64 and 65).
   // ************************************************************************************************************
   45: XIO(Command_Being_Processed)XIO(Local_Control.4)EQU(Type,2)GEQ(Converter.Command,15)LEQ(Converter.Command,16)OTL(Command_Being_Processed)MOV(Port,Port_Data.Data_Transfer[185])MOV(0,Port_Data.Data_Transfer[187])ADD(49,Converter.Command,Port_Data.Data_Transfer[188])MOV(2,Port_Data.Data_Transfer[189])SUB(Converter.Command,14,Index)OTL(Port_Data.Port_Read.[Port])OTL(Local_Control.4);
   46: XIO(Command_Being_Processed)XIO(Local_Control.4)XIO(Local_Control.6)NEQ(Type,2)GEQ(Converter.Command,15)LEQ(Converter.Command,16)OTU(Port_Data.Port_Read.[Port])OTL(Local_Control.6);
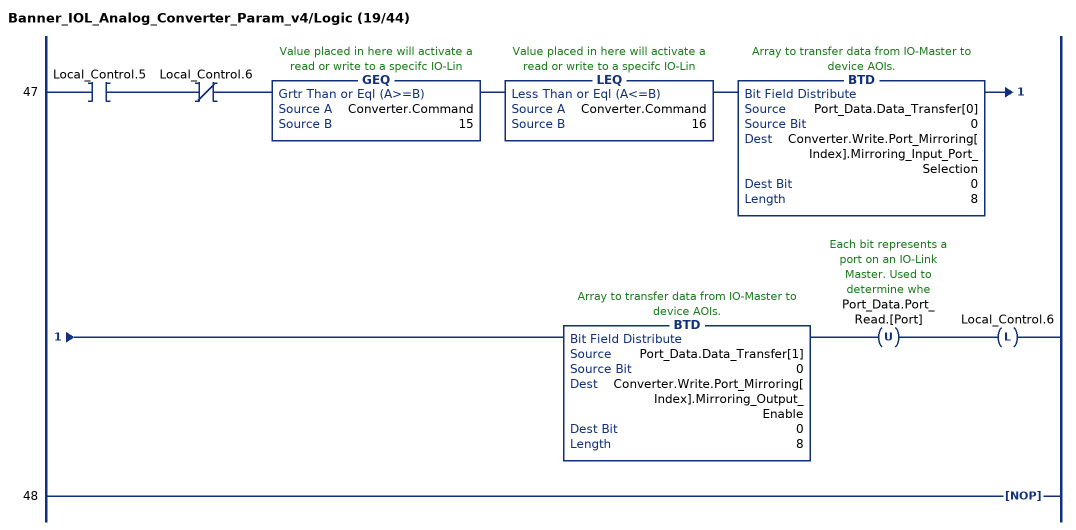
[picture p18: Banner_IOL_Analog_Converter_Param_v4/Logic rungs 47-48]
   47: XIC(Local_Control.5)XIO(Local_Control.6)GEQ(Converter.Command,15)LEQ(Converter.Command,16)BTD(Port_Data.Data_Transfer[0],0,Converter.Write.Port_Mirroring[Index].Mirroring_Input_Port_Selection,0,8)BTD(Port_Data.Data_Transfer[1],0,Converter.Write.Port_Mirroring[Index].Mirroring_Output_Enable,0,8)OTU(Port_Data.Port_Read.[Port])OTL(Local_Control.6);
   48: NOP();
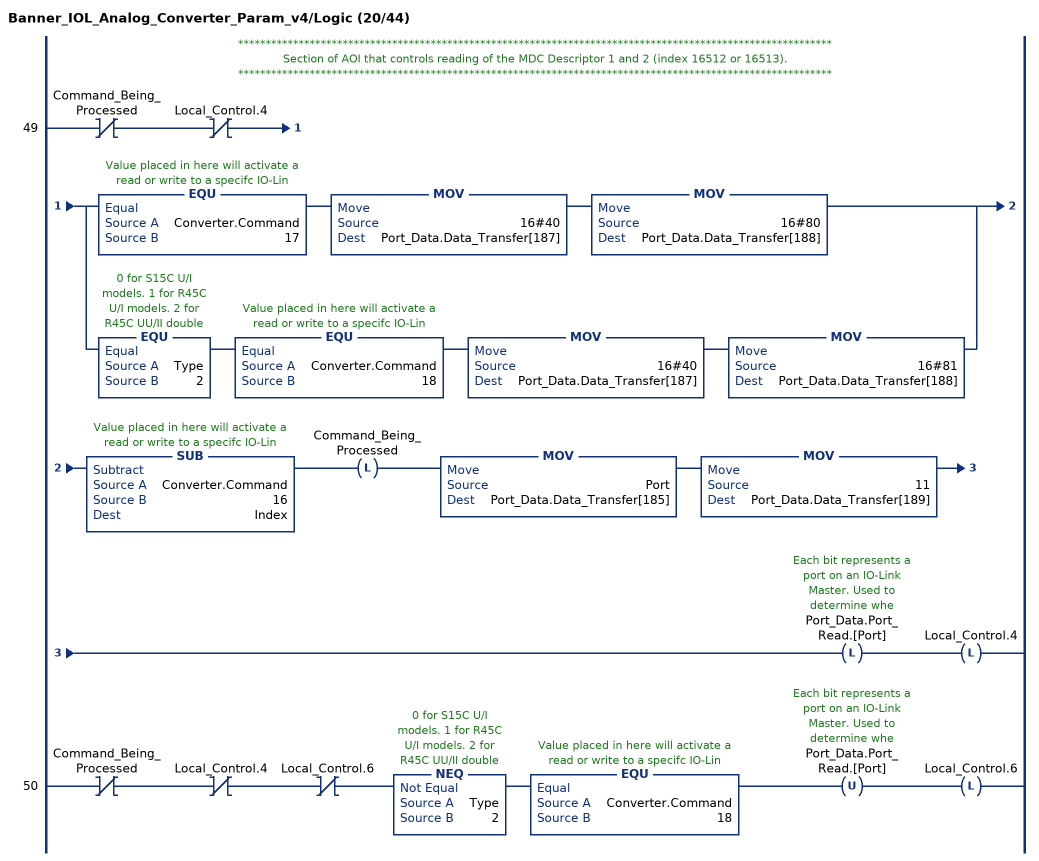
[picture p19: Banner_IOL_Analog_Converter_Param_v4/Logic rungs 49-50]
   // ************************************************************************************************************
   // Section of AOI that controls reading of the MDC Descriptor 1 and 2 (index 16512 or 16513).
   // ************************************************************************************************************
   49: XIO(Command_Being_Processed)XIO(Local_Control.4)[EQU(Converter.Command,17) MOV(16#40,Port_Data.Data_Transfer[187]) MOV(16#80,Port_Data.Data_Transfer[188]) ,EQU(Type,2) EQU(Converter.Command,18) MOV(16#40,Port_Data.Data_Transfer[187]) MOV(16#81,Port_Data.Data_Transfer[188]) ]SUB(Converter.Command,16,Index)OTL(Command_Being_Processed)MOV(Port,Port_Data.Data_Transfer[185])MOV(11,Port_Data.Data_Transfer[189])OTL(Port_Data.Port_Read.[Port])OTL(Local_Control.4);
   50: XIO(Command_Being_Processed)XIO(Local_Control.4)XIO(Local_Control.6)NEQ(Type,2)EQU(Converter.Command,18)OTU(Port_Data.Port_Read.[Port])OTL(Local_Control.6);
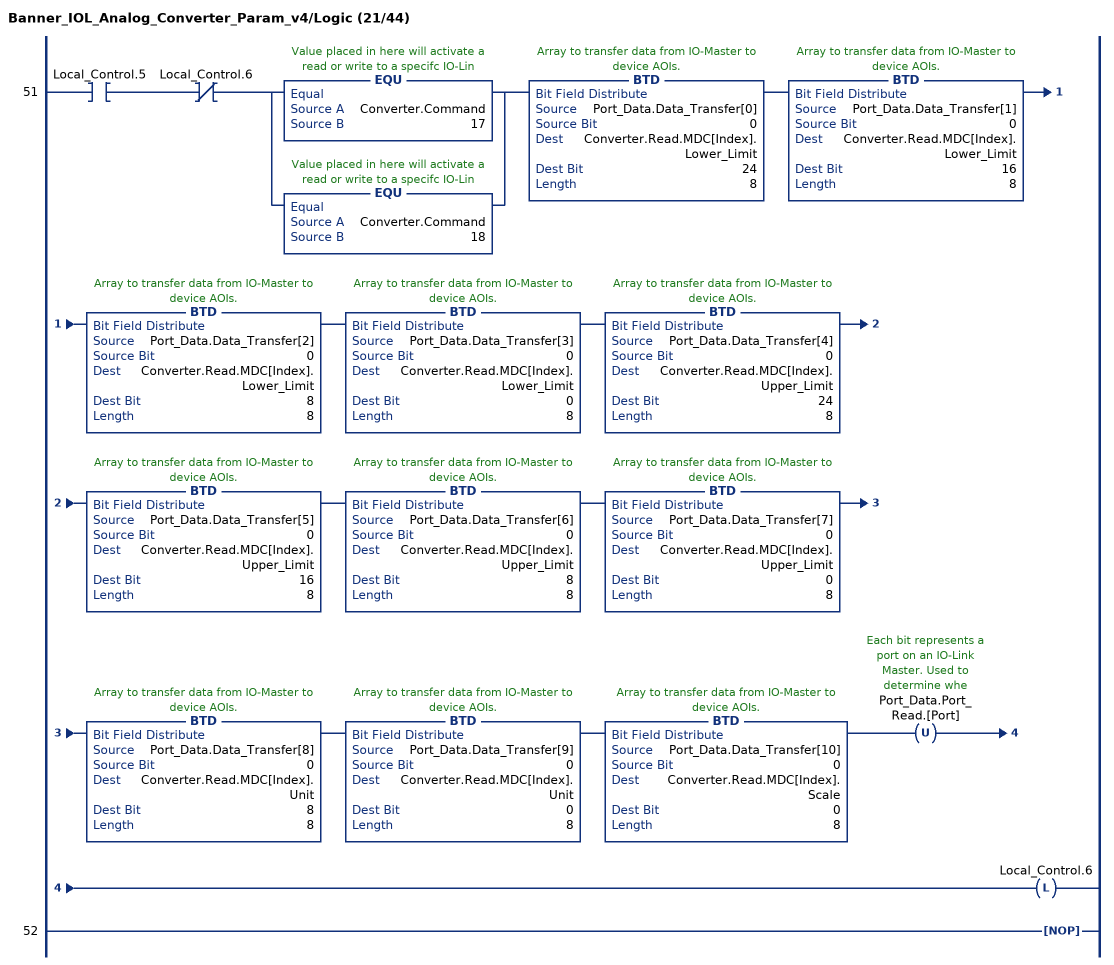
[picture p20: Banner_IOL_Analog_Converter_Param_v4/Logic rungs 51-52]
   51: XIC(Local_Control.5)XIO(Local_Control.6)[EQU(Converter.Command,17) ,EQU(Converter.Command,18) ]BTD(Port_Data.Data_Transfer[0],0,Converter.Read.MDC[Index].Lower_Limit,24,8)BTD(Port_Data.Data_Transfer[1],0,Converter.Read.MDC[Index].Lower_Limit,16,8)BTD(Port_Data.Data_Transfer[2],0,Converter.Read.MDC[Index].Lower_Limit,8,8)BTD(Port_Data.Data_Transfer[3],0,Converter.Read.MDC[Index].Lower_Limit,0,8)BTD(Port_Data.Data_Transfer[4],0,Converter.Read.MDC[Index].Upper_Limit,24,8)BTD(Port_Data.Data_Transfer[5],0,Converter.Read.MDC[Index].Upper_Limit,16,8)BTD(Port_Data.Data_Transfer[6],0,Converter.Read.MDC[Index].Upper_Limit,8,8)BTD(Port_Data.Data_Transfer[7],0,Converter.Read.MDC[Index].Upper_Limit,0,8)BTD(Port_Data.Data_Transfer[8],0,Converter.Read.MDC[Index].Unit,8,8)BTD(Port_Data.Data_Transfer[9],0,Converter.Read.MDC[Index].Unit,0,8)BTD(Port_Data.Data_Transfer[10],0,Converter.Read.MDC[Index].Scale,0,8)OTU(Port_Data.Port_Read.[Port])OTL(Local_Control.6);
   52: NOP();
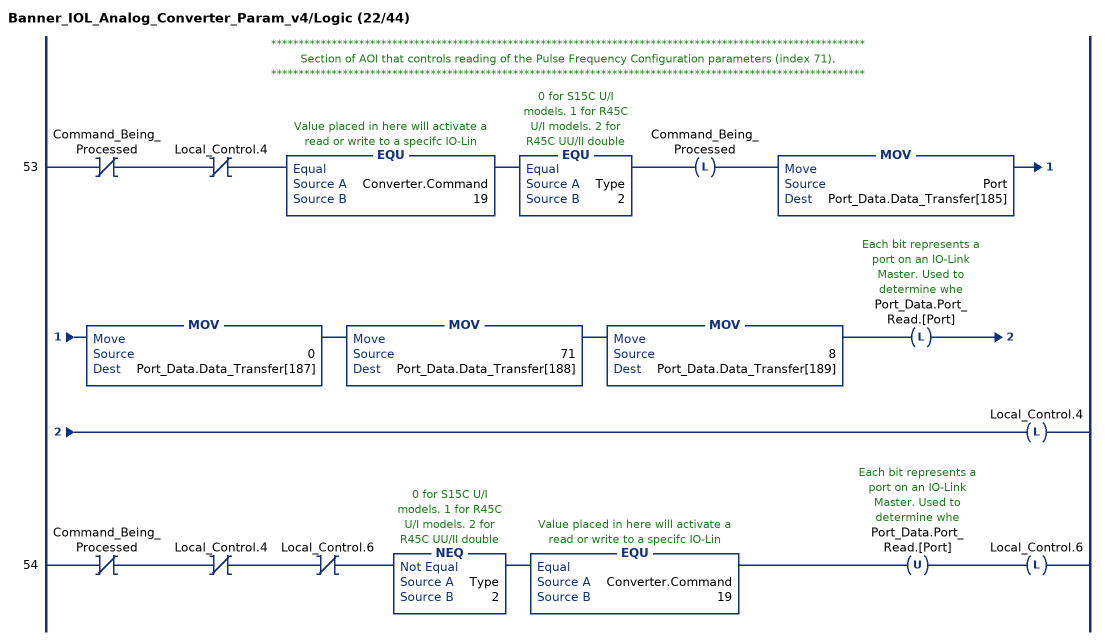
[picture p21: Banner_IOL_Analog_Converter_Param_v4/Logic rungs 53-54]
   // ************************************************************************************************************
   // Section of AOI that controls reading of the Pulse Frequency Configuration parameters (index 71).
   // ************************************************************************************************************
   53: XIO(Command_Being_Processed)XIO(Local_Control.4)EQU(Converter.Command,19)EQU(Type,2)OTL(Command_Being_Processed)MOV(Port,Port_Data.Data_Transfer[185])MOV(0,Port_Data.Data_Transfer[187])MOV(71,Port_Data.Data_Transfer[188])MOV(8,Port_Data.Data_Transfer[189])OTL(Port_Data.Port_Read.[Port])OTL(Local_Control.4);
   54: XIO(Command_Being_Processed)XIO(Local_Control.4)XIO(Local_Control.6)NEQ(Type,2)EQU(Converter.Command,19)OTU(Port_Data.Port_Read.[Port])OTL(Local_Control.6);
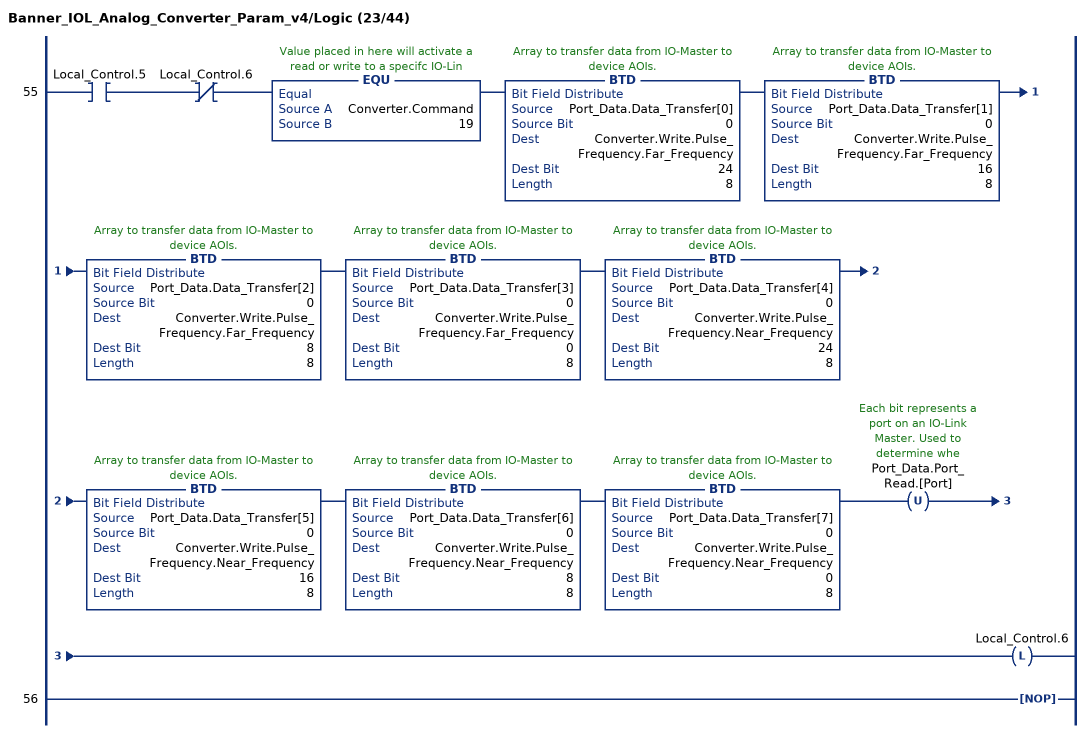
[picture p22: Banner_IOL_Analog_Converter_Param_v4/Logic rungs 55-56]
   55: XIC(Local_Control.5)XIO(Local_Control.6)EQU(Converter.Command,19)BTD(Port_Data.Data_Transfer[0],0,Converter.Write.Pulse_Frequency.Far_Frequency,24,8)BTD(Port_Data.Data_Transfer[1],0,Converter.Write.Pulse_Frequency.Far_Frequency,16,8)BTD(Port_Data.Data_Transfer[2],0,Converter.Write.Pulse_Frequency.Far_Frequency,8,8)BTD(Port_Data.Data_Transfer[3],0,Converter.Write.Pulse_Frequency.Far_Frequency,0,8)BTD(Port_Data.Data_Transfer[4],0,Converter.Write.Pulse_Frequency.Near_Frequency,24,8)BTD(Port_Data.Data_Transfer[5],0,Converter.Write.Pulse_Frequency.Near_Frequency,16,8)BTD(Port_Data.Data_Transfer[6],0,Converter.Write.Pulse_Frequency.Near_Frequency,8,8)BTD(Port_Data.Data_Transfer[7],0,Converter.Write.Pulse_Frequency.Near_Frequency,0,8)OTU(Port_Data.Port_Read.[Port])OTL(Local_Control.6);
   56: NOP();
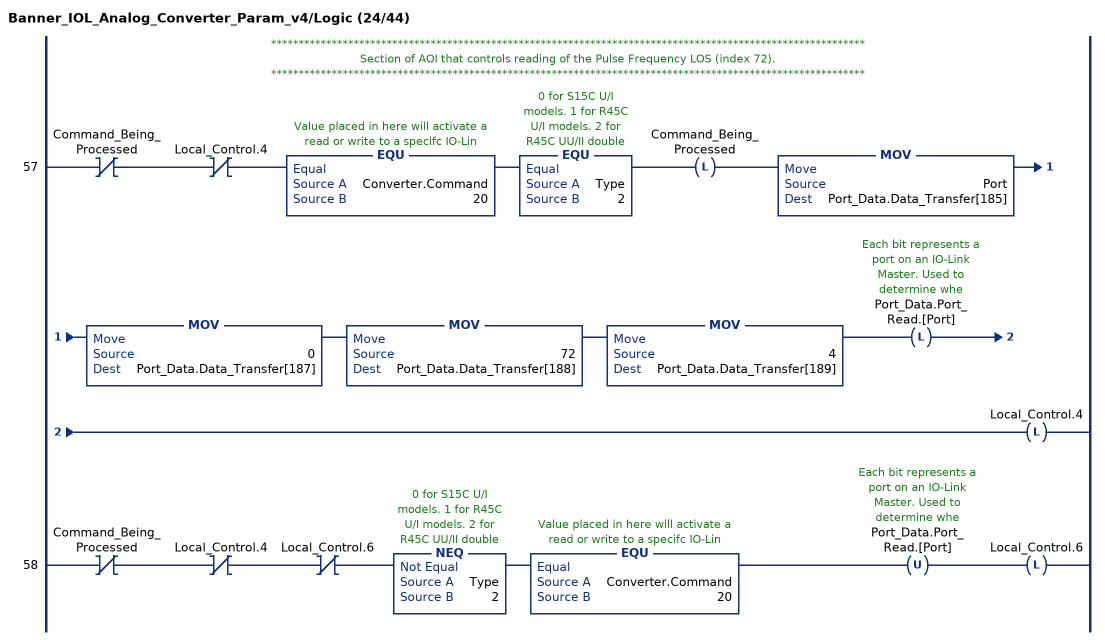
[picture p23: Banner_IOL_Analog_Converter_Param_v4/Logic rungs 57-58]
   // ************************************************************************************************************
   // Section of AOI that controls reading of the Pulse Frequency LOS (index 72).
   // ************************************************************************************************************
   57: XIO(Command_Being_Processed)XIO(Local_Control.4)EQU(Converter.Command,20)EQU(Type,2)OTL(Command_Being_Processed)MOV(Port,Port_Data.Data_Transfer[185])MOV(0,Port_Data.Data_Transfer[187])MOV(72,Port_Data.Data_Transfer[188])MOV(4,Port_Data.Data_Transfer[189])OTL(Port_Data.Port_Read.[Port])OTL(Local_Control.4);
   58: XIO(Command_Being_Processed)XIO(Local_Control.4)XIO(Local_Control.6)NEQ(Type,2)EQU(Converter.Command,20)OTU(Port_Data.Port_Read.[Port])OTL(Local_Control.6);
